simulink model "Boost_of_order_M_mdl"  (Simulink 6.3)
settings: Solver=ode45  StartTime=0.0  StopTime=10.0  RelTol=1e-6  AbsTol=1e-6
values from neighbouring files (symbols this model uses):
  Bg = ones(m,1)    [Boost_Duty_Cycle_R100.m]    (also in Boost_Duty_Cycle.m; Boost_of_order_M.m)
  C = 200*microF    (= 0.0002)    [Boost_Duty_Cycle_R100.m]    (also in Boost_Duty_Cycle.m; Boost_of_order_M.m)
  Duty_Cycle_m = Duty_Cycle([1:m])'    [Boost_of_order_M.m]
  Im_0 = 0*[1:m]'    [Boost_Duty_Cycle_R100.m]    (also in Boost_Duty_Cycle.m; Boost_of_order_M.m)
  Lm = eye(m)*L1    [Boost_Duty_Cycle_R100.m]    (also in Boost_Duty_Cycle.m; Boost_of_order_M.m = diag(L1m(1:m)))
  R = 100*Ohm    (= 100)    [Boost_Duty_Cycle_R100.m]    (also in Boost_Duty_Cycle.m = 19.9; Boost_of_order_M.m = 20)
  Rm = eye(m)*R1    [Boost_Duty_Cycle_R100.m]    (also in Boost_Duty_Cycle.m; Boost_of_order_M.m = diag(R1m(1:m)))
  Tc = Ts/50    (= 4e-07)    [Boost_Duty_Cycle_R100.m]    (also in Boost_Duty_Cycle.m; Boost_of_order_M.m)
  Ts = 0.02*msec    (= 2e-05)    [Boost_Duty_Cycle_R100.m]    (also in Boost_Duty_Cycle.m; Boost_of_order_M.m)
  Vc_0 = 0    [Boost_Duty_Cycle_R100.m]    (also in Boost_Duty_Cycle.m; Boost_of_order_M.m)
  Vg = 100*Volt    (= 100)    [Boost_Duty_Cycle_R100.m]    (also in Boost_Duty_Cycle.m; Boost_of_order_M.m)
libraries: simulink x1

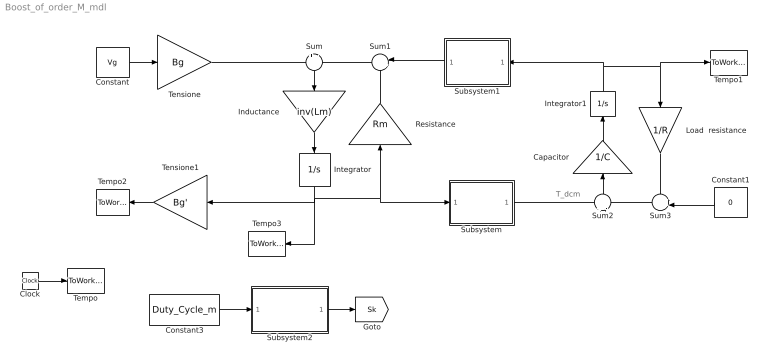
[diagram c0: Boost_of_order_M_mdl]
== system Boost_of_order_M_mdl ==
  note: T_dcm
  Capacitor : Gain  Orientation=up  Gain=1/C
  Clock : Clock
  Constant : Constant  Value=Vg
  Constant1 : Constant  Orientation=left  Value=0
  Constant3 : Constant  Value=Duty_Cycle_m
  Inductance : Gain  Orientation=down  Gain=inv(Lm)  Multiplication=Matrix(K*u) (u vector)
  Integrator : Integrator  Orientation=down  InitialCondition=Im_0  LimitOutput=on  LowerSaturationLimit=0
  Integrator1 : Integrator  Orientation=up  InitialCondition=Vc_0
  Load  resistance : Gain  Orientation=down  Gain=1/R
  Resistance : Gain  Orientation=up  Gain=Rm  Multiplication=Matrix(K*u) (u vector)
  Subsystem : Subsystem
  Subsystem1 : Subsystem  Orientation=left
  Subsystem2 : Subsystem
  Sum : Sum  Orientation=down  Inputs=+|-
  Sum1 : Sum  Orientation=left  Inputs=|++
  Sum2 : Sum  Orientation=up  Inputs=+|-
  Sum3 : Sum  Orientation=left  Inputs=++|
  Tempo : ToWorkspace  VariableName=t  SampleTime=Tc  SaveFormat=Array
  Tempo1 : ToWorkspace  VariableName=Vc  SampleTime=Tc  SaveFormat=Array
  Tempo2 : ToWorkspace  VariableName=Idc  SampleTime=Tc  SaveFormat=Array
  Tempo3 : ToWorkspace  VariableName=Im  SampleTime=Tc  SaveFormat=Array
  Tensione : Gain  Gain=Bg  Multiplication=Matrix(K*u) (u vector)
  Tensione1 : Gain  Orientation=left  Gain=Bg'  Multiplication=Matrix(K*u) (u vector)
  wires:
  Clock/1 -> Tempo/1
  Sum/1 -> Inductance/1
  Inductance/1 -> Integrator/1
  Integrator/1 -> Resistance/1, Subsystem/1(In1), Tempo3/1, Tensione1/1
  Sum1/1 -> Sum/2
  Resistance/1 -> Sum1/2
  Subsystem/1(Out1) -> Sum2/1
  Sum2/1 -> Capacitor/1
  Capacitor/1 -> Integrator1/1
  Integrator1/1 -> Load  resistance/1, Tempo1/1, Subsystem1/1(In1)
  Load  resistance/1 -> Sum3/1
  Sum3/1 -> Sum2/2
  Constant1/1 -> Sum3/2
  Subsystem1/1(Out1) -> Sum1/1
  Constant/1 -> Tensione/1
  Tensione/1 -> Sum/1
  Tensione1/1 -> Tempo2/1
  Subsystem2/1(Out1) -> [Sk]
  Constant3/1 -> Subsystem2/1(In1)

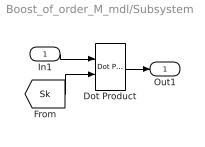
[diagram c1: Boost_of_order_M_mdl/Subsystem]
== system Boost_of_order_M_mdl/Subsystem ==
  In1 : Inport
  Dot Product : simulink/Math Operations/Dot Product  InputSameDT=on  OutDataType=sfix(16)  OutScaling=2^-10  DoSatur=off
  Out1 : Outport
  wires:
  [Sk] -> Dot Product/2
  In1/1 -> Dot Product/1
  Dot Product/1 -> Out1/1

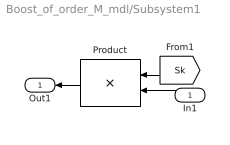
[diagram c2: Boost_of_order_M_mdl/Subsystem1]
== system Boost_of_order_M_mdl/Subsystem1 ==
  In1 : Inport  Orientation=left
  Product : Product  Orientation=left  Multiplication=Matrix(*)
  Out1 : Outport  Orientation=left
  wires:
  [Sk] -> Product/1
  In1/1 -> Product/2
  Product/1 -> Out1/1

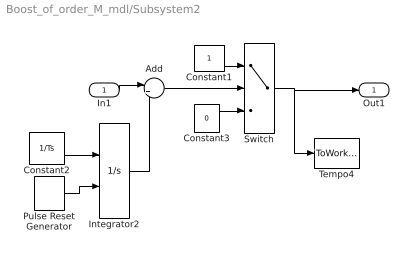
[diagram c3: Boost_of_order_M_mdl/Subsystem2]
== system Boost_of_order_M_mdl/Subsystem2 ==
  In1 : Inport
  Add : Sum  Inputs=|+-  OutScaling=2^-10
  Constant1 : Constant
  Constant2 : Constant  Value=1/Ts
  Constant3 : Constant  Value=0
  Integrator2 : Integrator  ExternalReset=rising
  Pulse Reset Generator : DiscretePulseGenerator  PulseType=Time based  Period=Ts  PulseWidth=50
  Switch : Switch
  Tempo4 : ToWorkspace  VariableName=S1  SampleTime=Tc  SaveFormat=Array
  Out1 : Outport
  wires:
  Pulse Reset Generator/1 -> Integrator2/2
  Constant2/1 -> Integrator2/1
  Integrator2/1 -> Add/2
  Add/1 -> Switch/2
  Switch/1 -> Tempo4/1, Out1/1
  In1/1 -> Add/1
  Constant1/1 -> Switch/1
  Constant3/1 -> Switch/3
